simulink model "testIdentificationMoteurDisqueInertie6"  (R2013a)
settings: Solver=ode45  StartTime=0  StopTime=1  FixedStep=1e-3  RelTol=1e-3  AbsTol=1e-4
PreLoadFcn:
  | warning('off','sm:sli:setup:compile:LocalSolverNotSupported')
model workspace (MAT data in the model file):
  handle : class17 (value not decoded)
  handle : class17 (value not decoded)
undefined symbols (not defined in the file or in its folder): kg, m, SimParam
libraries: MechanicalPartsLib x3, sm_lib x3, ElecDriverLib x1

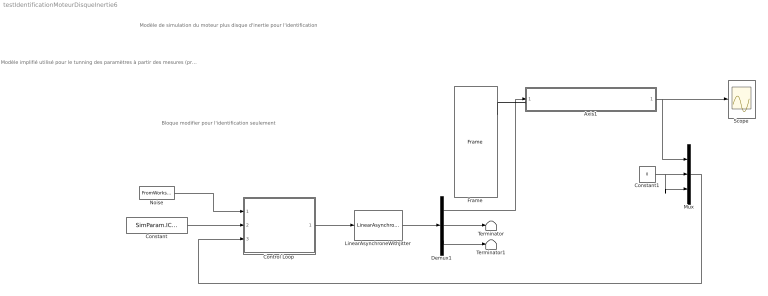
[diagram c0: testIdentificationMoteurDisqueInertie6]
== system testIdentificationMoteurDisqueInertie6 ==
  note: Bloque modifier pour l'identification seulement
  note: Modèle de simulation du moteur plus disque d'inertie pour l'identification
  note: Modèle implifié utilisé pour le tunning des paramètres à partir des mesures (prbs) effectuée sur le robot (Idem testIdentificationMoteur mais avec un élèment flexible dans le moteur) - Régulateur PID simple avec quantification codeur - Alimentation éléctrique modélisée par une fonction de transfert d'ordre deux avec delais (delais du contrôle) - Méchanique comprennant uniquement un modèle du moteur (inertie + frottement + 1ddl flexible en torsion) + frottement sec - Signaux d'exitation comprennant un bruit blanc et un signal cyclique (PRBS)
  Axis1 : Subsystem
  Constant : Constant  Value=SimParam.IC.Alpha
  Constant1 : Constant  Value=0
  Control Loop : Subsystem  Variant=on
  Demux1 : Demux  Outputs=3
  Frame : MechanicalPartsLib/Frame
  LinearAsynchroneWithJitter : ElecDriverLib/LinearAsynchroneWithJitter  VariantControl=driverVarLinearAsynchroneWithJitter
  Mux : Mux  Inputs=3
  Noise : FromWorkspace  VariableName=SimIn  SampleTime=SimParam.Control.Te  Interpolate=off  OutputAfterFinalValue=Holding final value
  Scope : Scope
  Terminator : Terminator
  Terminator1 : Terminator
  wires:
  Constant/1 -> Control Loop/2(Alpha_c)
  Mux/1 -> Control Loop/3(Alpha)
  Noise/1 -> Control Loop/1(Noise)
  Demux1/1 -> Axis1/1(Torque)
  LinearAsynchroneWithJitter/1 -> Demux1/1
  Control Loop/1(U) -> LinearAsynchroneWithJitter/1
  Axis1/1(Alpha) -> Mux/1, Scope/1
  Constant1/1 -> Mux/3, Mux/2
  Demux1/2 -> Terminator/1
  Demux1/3 -> Terminator1/1
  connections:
  Frame/RConn1 -- Axis1/LConn1

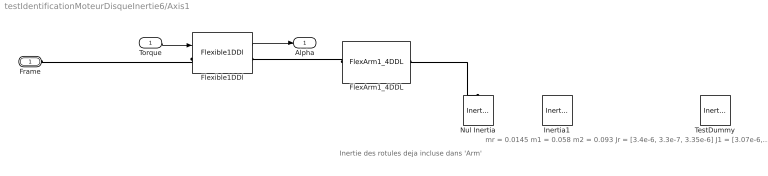
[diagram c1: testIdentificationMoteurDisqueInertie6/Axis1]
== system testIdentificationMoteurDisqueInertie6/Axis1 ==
  note: Inertie des rotules deja incluse dans 'Arm'
  note: mr = 0.0145 m1 = 0.058 m2 = 0.093 Jr = [3.4e-6, 3.3e-7, 3.35e-6] J1 = [3.07e-6, 4.18e-6, 5.04e-6] J2 = [6.29e-6, 10.2e-6, 10.2e-6]
  Torque : Inport
  FlexArm1_4DDL : MechanicalPartsLib/FlexArm1_4DDL  VariantControl=armVarFlex1_4ddl
  Flexible1DDl : MechanicalPartsLib/Flexible1DDl  VariantControl=motorVarFlex1
  Inertia1 : sm_lib/Body Elements/Inertia  Commented=on  InertiaType=Custom  Mass=0.083  MassUnits=kg  CenterOfMass=[0 0 0]  CenterOfMassUnits=m  MomentsOfInertia=[6.29e-6, 10.2e-6, 10.2e-6]  MomentsOfInertiaUnits=kg*m^2  ProductsOfInertia=[0 0 0]  ProductsOfInertiaUnits=kg*m^2  BlockFunction=simmechanics.library.body_elements.inertia
  Nul Inertia : sm_lib/Body Elements/Inertia  InertiaType=Custom  Mass=1e-5  MassUnits=kg  CenterOfMass=[0 0 0]  CenterOfMassUnits=m  MomentsOfInertia=[1e-8 1e-8 1e-8]  MomentsOfInertiaUnits=kg*m^2  ProductsOfInertia=[0 0 0]  ProductsOfInertiaUnits=kg*m^2  BlockFunction=simmechanics.library.body_elements.inertia
  TestDummy : sm_lib/Body Elements/Inertia  Commented=on  InertiaType=Custom  Mass=0.0145  MassUnits=kg  CenterOfMass=[0 0 0]  CenterOfMassUnits=m  MomentsOfInertia=[3.4e-6, 3.3e-7, 3.35e-6]  MomentsOfInertiaUnits=kg*m^2  ProductsOfInertia=[0 0 0]  ProductsOfInertiaUnits=kg*m^2  BlockFunction=simmechanics.library.body_elements.inertia
  Frame : PMIOPort  Port=1  Side=Left
  Alpha : Outport
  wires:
  Torque/1 -> Flexible1DDl/1
  Flexible1DDl/1 -> Alpha/1
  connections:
  FlexArm1_4DDL/RConn1 -- Nul Inertia/RConn1
  FlexArm1_4DDL/LConn1 -- Flexible1DDl/RConn1
  Flexible1DDl/LConn1 -- Frame/RConn1

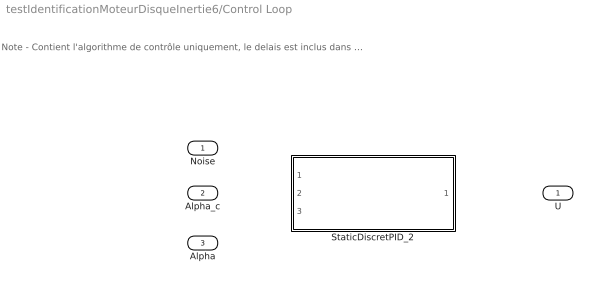
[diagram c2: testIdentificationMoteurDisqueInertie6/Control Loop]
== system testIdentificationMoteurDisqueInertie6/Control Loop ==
  note: Note - Contient l'algorithme de contrôle uniquement, le delais est inclus dans le bloque 'Electric Drive'
  Noise : Inport
  Alpha_c : Inport  Port=2
  Alpha : Inport  Port=3
  StaticDiscretPID_2 : Subsystem  VariantControl=controlVarDefault
  U : Outport

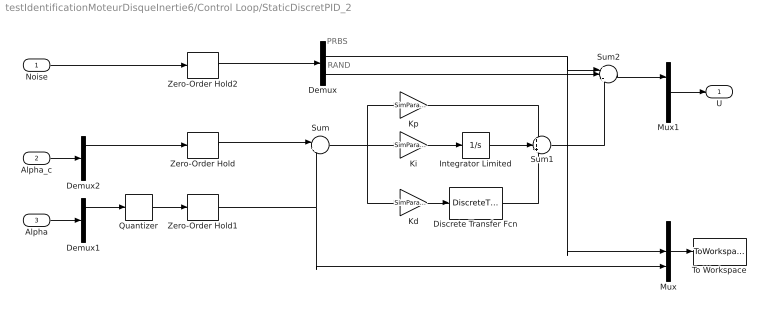
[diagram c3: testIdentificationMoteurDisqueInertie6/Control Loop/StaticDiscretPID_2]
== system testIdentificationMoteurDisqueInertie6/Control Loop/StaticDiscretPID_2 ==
  note: RAND
  note: PRBS
  Noise : Inport
  Alpha_c : Inport  Port=2
  Alpha : Inport  Port=3
  Demux : Demux  Outputs=2
  Demux1 : Demux  Outputs=3
  Demux2 : Demux  Outputs=3
  Discrete Transfer Fcn : DiscreteTransferFcn  Numerator=[1 0 -1]  Denominator=[2 0 0]
  Integrator Limited : Integrator  LimitOutput=on  UpperSaturationLimit=1  LowerSaturationLimit=-1
  Kd : Gain  Gain=SimParam.Control.Kd/SimParam.Control.Te
  Ki : Gain  Gain=SimParam.Control.Ki*SimParam.Control.Te
  Kp : Gain  Gain=SimParam.Control.Kp
  Mux : Mux  Inputs=3
  Mux1 : Mux  Inputs=3
  Quantizer : Quantizer  QuantizationInterval=2*pi/(4500*4*25)
  Sum : Sum  Inputs=|+-
  Sum1 : Sum  Inputs=+++
  Sum2 : Sum  Inputs=+++
  To Workspace : ToWorkspace  VariableName=simout  SampleTime=SimParam.Control.Te  SaveFormat=Structure With Time
  Zero-Order Hold : ZeroOrderHold  SampleTime=SimParam.Control.Te
  Zero-Order Hold1 : ZeroOrderHold  SampleTime=SimParam.Control.Te
  Zero-Order Hold2 : ZeroOrderHold  SampleTime=SimParam.Control.Te
  U : Outport
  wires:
  Kd/1 -> Discrete Transfer Fcn/1
  Mux/1 -> To Workspace/1
  Zero-Order Hold/1 -> Sum/1
  Quantizer/1 -> Zero-Order Hold1/1
  Noise/1 -> Zero-Order Hold2/1
  Discrete Transfer Fcn/1 -> Sum1/3
  Kp/1 -> Sum1/1
  Sum1/1 -> Sum2/3
  Demux/1 -> Mux/2, Sum2/1
  Ki/1 -> Integrator Limited/1
  Integrator Limited/1 -> Sum1/2
  Sum/1 -> Ki/1, Kp/1, Kd/1
  Zero-Order Hold1/1 -> Mux/3, Sum/2
  Demux/2 -> Sum2/2
  Zero-Order Hold2/1 -> Demux/1
  Demux1/1 -> Quantizer/1
  Alpha/1 -> Demux1/1
  Demux2/1 -> Zero-Order Hold/1
  Alpha_c/1 -> Demux2/1
  Mux1/1 -> U/1
  Sum2/1 -> Mux1/1
